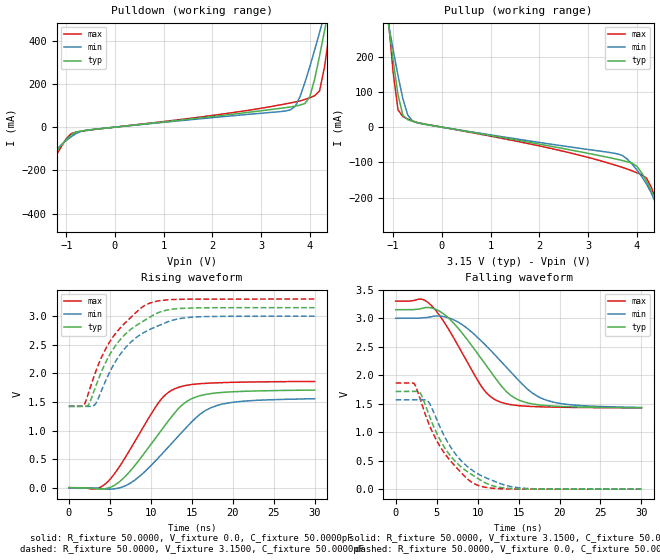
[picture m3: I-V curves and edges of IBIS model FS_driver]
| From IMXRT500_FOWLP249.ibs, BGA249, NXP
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[Model] FS_driver
|   Model FS_driver
| Library cells for typ/min/max conditions are connected as defined below:
|  pad_usbdp - External Pad
|  usb2_tx_d_data_dp - Core Input
|  gnda - gnda
|  pad_usb_vss - pad_usb_vss
|  usb2_reg_tx_fs_hiz - gnda
|  usb2_reg_tx_hs_term - gnda
|  usb2_reg_tx_hs_xcvr - gnda
|  usb2_reg_tx_ls_en - gnda
|  usbphy_d2a_txhsactive - gnda
|  vddb - vddb
|  vddd - vddd
| All other pins connected to ground
Model_type Output
Polarity   Non-Inverting
Enable   Active-Low
C_comp   2.8431pF   2.6338pF   3.0727pF
[Temperature Range]   27.0000   0.1250k   -40.0000
[Voltage Range]   3.1500V   3.0000V   3.3000V
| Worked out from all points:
|   slope of the pulldown table from 0 to 0.472 V, typ, clamps not added: 41.5 ohm
|   slope of the pullup table from 0 to 0.472 V, typ, clamps not added: 42.2 ohm
|   rising waveform, R_fixture 50.0000, V_fixture 0.0, C_fixture 50.0000pF: 20-80 % time 5.48ns typ, 6.19ns min, 4.75ns max; typ from 0 V to 1.71 V
|   rising waveform, R_fixture 50.0000, V_fixture 3.1500, C_fixture 50.0000pF: 20-80 % time 4.62ns typ, 4.72ns min, 4.45ns max; typ from 1.42 V to 3.15 V
|   falling waveform, R_fixture 50.0000, V_fixture 3.1500, C_fixture 50.0000pF: 20-80 % time 5.39ns typ, 6.32ns min, 4.53ns max; typ from 3.15 V to 1.43 V
|   falling waveform, R_fixture 50.0000, V_fixture 0.0, C_fixture 50.0000pF: 20-80 % time 4.52ns typ, 4.62ns min, 4.26ns max; typ from 1.72 V to 0 V
[Pulldown]
|Voltage   I(typ)   I(min)   I(max)
-3.3V     -1.789A    -1.328A    -2.415A
-2V       -541mA     -458.4mA   -672.7mA
-1.8V     -385mA     -344.5mA   -475.2mA
-1.2V     -110.9mA   -103.2mA   -128.7mA
-700mV    -18.35mA   -19.33mA   -19.54mA
3.6V      93.13mA    79.46mA    111.7mA
4V        140.3mA    280mA      135.9mA
4.2V      328.8mA    437.3mA    167.5mA
4.3V      443.1mA    519.1mA    276.2mA
4.4V      562.1mA    602.3mA    433.8mA
4.5V      683.9mA    686.7mA    605.7mA
6.6V      3.469A     2.552A     4.733A
[Pullup]
|Voltage   I(typ)   I(min)   I(max)
-3.3V     3.149A     2.232A     4.536A
-1.1V     298.4mA    297.3mA    309.5mA
-1V       188.4mA    219.5mA    155mA
-900mV    91.83mA    145.9mA    49.27mA
-800mV    33.62mA    80.51mA    29.57mA
-700mV    21.24mA    34.27mA    23.01mA
-400mV    9.525mA    9.075mA    10.13mA
3.7V      -94.61mA   -80.02mA   -113.9mA
4V        -110.4mA   -120.8mA   -129.3mA
4.2V      -153.7mA   -161.4mA   -144.6mA
4.6V      -279.6mA   -298.9mA   -297.9mA
6.6V      -2.055A    -1.587A    -2.608A
[Ramp]
| variable   typ   min   max
dV/dt_r  0.9764/5.3405n   0.8872/6.0434n   1.0659/4.5928n
dV/dt_f  0.9849/5.2520n   0.8928/6.1804n   1.0738/4.3755n
R_load = 45.0000
[Rising Waveform]
R_fixture= 50.0000
V_fixture= 0.0
V_fixture_min= 0.0
V_fixture_max= 0.0
C_fixture= 50.0000pF
|time   V(typ)   V(min)   V(max)
0s        96.56nV    2.993uV    69.84nV
3.224ns   -18.2mV    -5.747mV   -19.86mV
4.678ns   -11.17mV   -24.86mV   94.38mV
6.235ns   109.8mV    -1.054mV   379.3mV
8.045ns   386mV      131.9mV    806.6mV
11.17ns   982.7mV    557.9mV    1.528V
12.97ns   1.316V     841mV      1.732V
14.93ns   1.552V     1.141V     1.803V
18.12ns   1.659V     1.439V     1.835V
30ns      1.708V     1.556V     1.859V
[Rising Waveform]
R_fixture= 50.0000
V_fixture= 3.1500
V_fixture_min= 3.0000
V_fixture_max= 3.3000
C_fixture= 50.0000pF
|time   V(typ)   V(min)   V(max)
0s        1.422V     1.421V     1.425V
1.83ns    1.422V     1.421V     1.44V
2.448ns   1.46V      1.421V     1.679V
3.181ns   1.734V     1.453V     1.992V
4.457ns   2.18V      1.858V     2.418V
5.922ns   2.528V     2.26V      2.737V
7.517ns   2.764V     2.539V     2.971V
9.727ns   2.969V     2.757V     3.22V
14.92ns   3.144V     2.982V     3.298V
30ns      3.149V     2.999V     3.3V
[Falling Waveform]
R_fixture= 50.0000
V_fixture= 3.1500
V_fixture_min= 3.0000
V_fixture_max= 3.3000
C_fixture= 50.0000pF
|time   V(typ)   V(min)   V(max)
0s        3.15V      3V         3.3V
3.106ns   3.171V     3.004V     3.336V
4.315ns   3.184V     3.026V     3.231V
5.898ns   3.071V     3.029V     2.936V
7.845ns   2.788V     2.913V     2.461V
10.76ns   2.228V     2.559V     1.746V
12.51ns   1.883V     2.296V     1.545V
14.92ns   1.572V     1.924V     1.468V
18.5ns    1.465V     1.556V     1.442V
30ns      1.428V     1.435V     1.428V
[Falling Waveform]
R_fixture= 50.0000
V_fixture= 0.0
V_fixture_min= 0.0
V_fixture_max= 0.0
C_fixture= 50.0000pF
|time   V(typ)   V(min)   V(max)
0s        1.715V     1.569V     1.863V
2.271ns   1.717V     1.569V     1.85V
3.004ns   1.685V     1.571V     1.573V
3.916ns   1.362V     1.546V     1.194V
6.46ns    627mV      796.3mV    535.4mV
8.065ns   381.7mV    488.7mV    278.1mV
9.918ns   198.2mV    279.1mV    73.97mV
12.07ns   50.47mV    136.5mV    13.58mV
15.63ns   3.695mV    16.32mV    1.07mV
30ns      185.1uV    307.2uV    126.6uV
